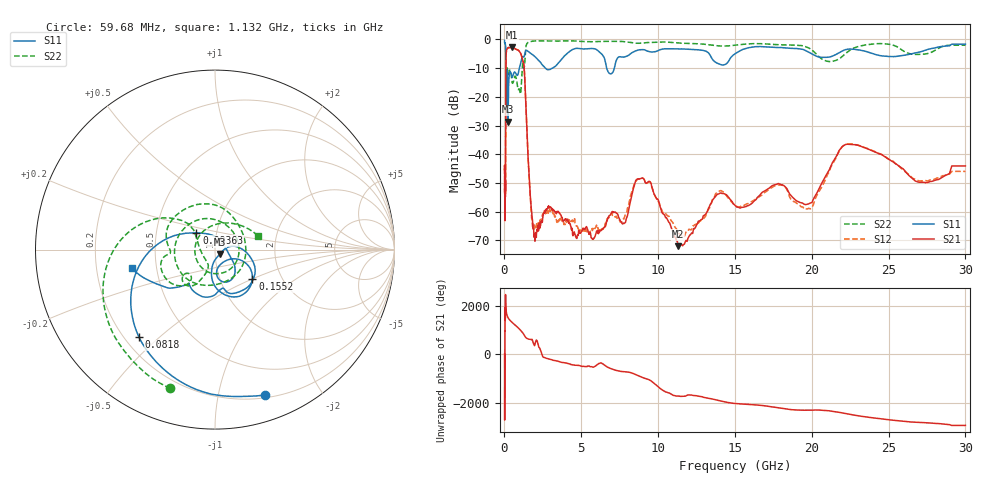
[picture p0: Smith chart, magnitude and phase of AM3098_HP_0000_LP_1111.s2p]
! Date/Time: Thu, Feb 28, 2019 8:31 AM
! Network Analyzer: Agilent Technologies E8364B Rev: A.07.50.67
! Sweep from 0.010 to 30.000 GHz, 1601 Points, Sweep Type: LOG
! Power Supply: 5.022 V, 0.002 A
# Hz S DB R 50
!freq MagS11 AngS11 MagS21 AngS21 MagS12 AngS12 MagS22 AngS22
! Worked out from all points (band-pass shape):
!   1601 points, 10 MHz to 30 GHz, reference 50 ohm
!   highest |S21| = -2.75 dB at 498 MHz (marker M1); lowest = -72.0 dB at 11.31 GHz (marker M2)
!   |S21| within 3 dB of the highest: 105.1 MHz to 1.113 GHz (1.008 GHz wide, 165 % of centre)
!   lowest |S11| = -28.6 dB at 231.6 MHz (marker M3), VSWR 1.08, Z = 52.8 - j2.56 ohm
!   |S11| at or under -10 dB: 90.4 MHz to 972.7 MHz (882.3 MHz wide, 166 % of centre); 2.666 GHz to 3.135 GHz (468.2 MHz wide, 16.1 % of centre); 6.653 GHz to 7.15 GHz (497 MHz wide, 7.2 % of centre)
!   |S22| runs from -22.6 to -0.5 dB; largest |S21 - S12| = 0.011
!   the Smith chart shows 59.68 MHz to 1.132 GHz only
!   S11 on the Smith chart (normalised r, x): 59.68 MHz: 0.23, -1.37; 81.8 MHz: 0.26, -0.43; 93.63 MHz: 0.80, +0.15; 155.2 MHz: 1.42, -0.51; 1.132 GHz: 0.36, -0.10
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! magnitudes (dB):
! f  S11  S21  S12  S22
! 10 MHz  -0.4  -45.4  -45.5  -0.6
! 38.04 MHz  -0.5  -60.0  -58.6  -1.1
! 59.68 MHz  -1.4  -49.2  -50.6  -1.8
! 70.04 MHz  -1.9  -51.8  -51.5  -2.4
! 81.8 MHz  -3.8  -33.0  -32.8  -4.2
! 93.63 MHz  -17.1  -11.3  -11.3  -20.8
! 144.7 MHz  -14.2  -3.5  -3.4  -12.7
! 155.2 MHz  -11.5  -3.4  -3.4  -11.0
! 231.6 MHz  -28.6  -2.9  -2.9  -12.0
! 498 MHz  -13.2  -2.8  -2.7  -14.9
! 550.5 MHz  -12.6  -2.9  -2.9  -15.1
! 1.132 GHz  -6.5  -6.1  -6.1  -12.0
! 1.308 GHz  -5.4  -12.2  -12.1  -8.9
! 1.784 GHz  -5.1  -61.3  -63.3  -0.6
! 2.084 GHz  -6.5  -67.6  -64.8  -0.5
! 7.926 GHz  -5.9  -62.5  -60.8  -0.9
! 9.164 GHz  -3.7  -49.8  -49.9  -1.1
! 11.31 GHz  -3.3  -72.0  -67.5  -1.2
! 14.02 GHz  -8.7  -53.6  -52.8  -2.3
! 19.61 GHz  -3.9  -57.6  -59.0  -2.5
! 22.67 GHz  -3.4  -36.6  -36.4  -3.2
! 30 GHz  -1.7  -44.1  -46.0  -2.0
